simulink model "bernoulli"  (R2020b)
settings: Solver=VariableStepAuto  StartTime=0.0  StopTime=20.0  RelTol=1e-3
model workspace (MAT data in the model file):
  L = 3
  g = 9.81
  h = 1
  hx = 1.3
  p = 100000
  rho = 997

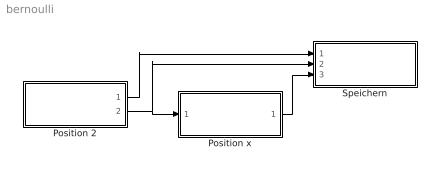
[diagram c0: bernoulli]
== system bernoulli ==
  Position 2 : Subsystem
  Position x : Subsystem
  Speichern : Subsystem
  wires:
  Position 2/2(a2) -> Position x/1(a2), Speichern/2(a2)
  Position 2/1(v2) -> Speichern/1(v2)
  Position x/1(px) -> Speichern/3(px)

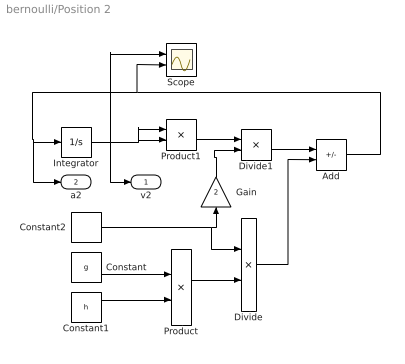
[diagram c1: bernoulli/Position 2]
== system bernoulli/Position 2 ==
  Add : Sum  Inputs=-+
  Constant : Constant  Value=g
  Constant1 : Constant  Value=h
  Constant2 : Constant  Value=L
  Divide : Product  Inputs=/*
  Divide1 : Product  Inputs=*/
  Gain : Gain  Gain=2
  Integrator : Integrator
  Product : Product
  Product1 : Product
  Scope : Scope  NumInputPorts=2
  v2 : Outport
  a2 : Outport  Port=2
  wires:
  Constant/1 -> Product/1
  Constant1/1 -> Product/2
  Product/1 -> Divide/2
  Constant2/1 -> Divide/1, Gain/1
  Divide/1 -> Add/2
  Integrator/1 -> Scope/1, v2/1, Product1/2, Product1/1
  Product1/1 -> Divide1/1
  Gain/1 -> Divide1/2
  Divide1/1 -> Add/1
  Add/1 -> Scope/2, a2/1, Integrator/1

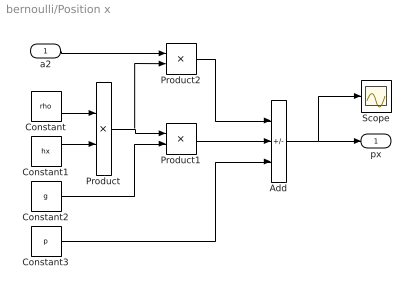
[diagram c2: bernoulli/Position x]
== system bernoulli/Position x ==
  a2 : Inport
  Add : Sum  Inputs=+-+
  Constant : Constant  Value=rho
  Constant1 : Constant  Value=hx
  Constant2 : Constant  Value=g
  Constant3 : Constant  Value=p
  Product : Product
  Product1 : Product
  Product2 : Product
  Scope : Scope
  px : Outport
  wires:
  Constant/1 -> Product/1
  Constant1/1 -> Product/2
  Product/1 -> Product2/2, Product1/1
  Constant2/1 -> Product1/2
  a2/1 -> Product2/1
  Constant3/1 -> Add/3
  Product1/1 -> Add/2
  Product2/1 -> Add/1
  Add/1 -> Scope/1, px/1

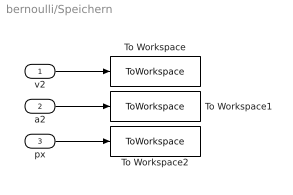
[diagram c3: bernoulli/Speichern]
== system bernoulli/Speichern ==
  v2 : Inport
  a2 : Inport  Port=2
  px : Inport  Port=3
  To Workspace : ToWorkspace  VariableName=v2  SaveFormat=Timeseries  SampleTime=-1
  To Workspace1 : ToWorkspace  VariableName=a2  SaveFormat=Timeseries  SampleTime=-1
  To Workspace2 : ToWorkspace  VariableName=px  SaveFormat=Timeseries  SampleTime=-1
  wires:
  v2/1 -> To Workspace/1
  a2/1 -> To Workspace1/1
  px/1 -> To Workspace2/1
